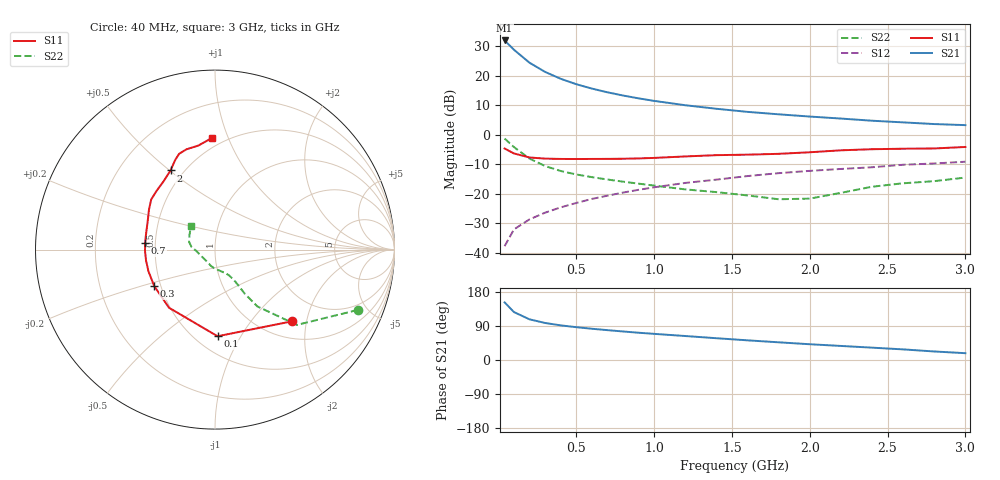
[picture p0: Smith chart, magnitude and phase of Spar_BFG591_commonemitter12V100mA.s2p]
! Filename:  BFG591J.S2P  Version:  4.0
! NXP part #: BFG591  Date: Jun 1994
! Bias condition: Vce=12V; Ic=100mA
#  MHz  S  MA  R  50
! Freq  S11  S21  S12  S22  !GUM [dB]
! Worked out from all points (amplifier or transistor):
!   21 points, 40 MHz to 3 GHz, reference 50 ohm
!   highest |S21| = 32.0 dB at 40 MHz (marker M1)
!   |S21| within 3 dB of that: start of sweep to 97.42 MHz
!   unconditionally stable (mu >= 1): 589.1 MHz to 2.174 GHz
!   at 300 MHz: K = 0.85, MSG = 23.8 dB, |S12| = -26.4 dB
!   at 1 GHz: K = 1.05, MAG = 13.3 dB, |S12| = -17.8 dB
!   at 3 GHz: K = 0.95, MSG = 6.2 dB, |S12| = -9.1 dB
!   S11 on the Smith chart (normalised r, x): 40 MHz: 1.35, -1.64; 100 MHz: 0.64, -0.80; 300 MHz: 0.46, -0.22; 700 MHz: 0.44, +0.04; 2 GHz: 0.42, +0.50; 3 GHz: 0.43, +0.87
40  0.586 -43.0  39.59 152.1  0.013 71.7  0.864 -22.9
100  0.483 -88.3  27.6 126.5  0.025 61.5  0.62 -42.6
200  0.413 -128.3  16.61 107.3  0.037 60.2  0.395 -53.3
300  0.395 -149.0  11.62 97.7  0.048 62.5  0.296 -56.0
400  0.39 -162.0  8.886 91.4  0.059 64.8  0.244 -56.8
500  0.389 -171.2  7.192 86.6  0.07 66.2  0.213 -57.6
600  0.39 -178.8  6.069 82.5  0.082 66.7  0.192 -58.7
700  0.391 174.9  5.246 78.8  0.093 67.2  0.175 -60.1
800  0.393 168.8  4.631 75.3  0.105 67.2  0.161 -61.9
900  0.398 162.8  4.145 72.0  0.117 67.2  0.149 -64.7
1000  0.406 157.6  3.753 69.0  0.129 66.7  0.138 -68.4
1200  0.43 148.8  3.169 63.3  0.153 65.3  0.119 -78.3
1400  0.452 141.9  2.76 57.5  0.174 63.4  0.107 -90.2
1600  0.461 135.2  2.446 51.9  0.2 62.1  0.094 -103.6
1800  0.476 127.1  2.223 46.7  0.224 59.0  0.081 -121.9
2000  0.506 119.3  2.037 41.6  0.245 57.1  0.083 -152.1
2200  0.546 114.0  1.884 37.1  0.264 54.9  0.104 -175.6
2400  0.57 110.5  1.732 32.6  0.282 53.9  0.132 173.4
2600  0.581 105.9  1.623 28.0  0.311 50.2  0.151 163.3
2800  0.587 99.1  1.52 22.5  0.327 46.2  0.164 150.1
3000  0.622 91.6  1.458 18.0  0.35 44.7  0.189 135.0
